[IBIS Ver]   3.2
[Comment Char]   |_char
[File Name]   sprm301.ibs
[File Rev]   1.0
[Date]   November 15, 2006
[Source]   From Ansoft Q3D ver 7.0 result.
[Notes]
[Disclaimer]
[Copyright]
[Component]   F28044PZ
[Manufacturer]   ti
[Package]
| variable   typ   min   max
R_pkg   2.03359e-001  1.85676e-001  2.33646e-001
L_pkg   4.42275e-009  3.91388e-009  5.16902e-009
C_pkg   6.90400e-013  6.03899e-013  7.98201e-013
[Pin]  signal_name   model_name   R_pin   L_pin   C_pin
01   GP_IO[12]  BC3350AFHYPU_3P3PU   2.16292E-01  4.84246E-09  7.01525E-13
02   VSS   NC   2.05669E-01  4.59853E-09  7.81026E-13
03   VDDIO   NC   2.14427E-01  4.64717E-09  7.53822E-13
04   GP_IO[29]  BC3325CFHYPU_3P3PU   2.26264E-01  4.68911E-09  7.55451E-13
05   GP_IO[33]  BC3350AFHYPU_3P3PU   2.15510E-01  4.52774E-09  7.45637E-13
06   GP_IO[30]  BC3325CFHYPU_3P3PU   2.05271E-01  4.36673E-09  7.14612E-13
07   GP_IO[31]  BC3325CFHYPU_3P3PU   2.01452E-01  4.28833E-09  6.88677E-13
08   GP_IO[14]  BC3350AFHYPU_3P3PU   1.93969E-01  4.17968E-09  6.67444E-13
09   GP_IO[15]  BC3350AFHYPU_3P3PU   1.92673E-01  4.14893E-09  6.50213E-13
10   VDD   NC   1.88856E-01  4.10765E-09  6.26914E-13
11   VSS   NC   1.92989E-01  4.13681E-09  6.03899E-13
12   VDD1   NC   2.13333E-01  4.32411E-09  6.20891E-13
13   VSS1   NC   2.06448E-01  4.25241E-09  6.31248E-13
14   VSSA2   NC   2.00063E-01  4.20609E-09  6.23019E-13
15   VDDAFL2   NC   1.93798E-01  4.16585E-09  6.28937E-13
16   ADCINA[7]   NC   1.89234E-01  4.18448E-09  6.36262E-13
17   ADCINA[6]   NC   1.87412E-01  4.23464E-09  6.46472E-13
18   ADCINA[5]   NC   1.86137E-01  4.27562E-09  6.59873E-13
19   ADCINA[4]   NC   1.85769E-01  4.34569E-09  6.75681E-13
20   ADCINA[3]   NC   1.87173E-01  4.42449E-09  6.94435E-13
21   ADCINA[2]   NC   1.89523E-01  4.53444E-09  7.11496E-13
22   ADCINA[1]   NC   1.93470E-01  4.65439E-09  7.32914E-13
23   ADCINA[0]   NC   1.96936E-01  4.78656E-09  7.54045E-13
24   ADCLO   NC   2.02141E-01  4.91416E-09  7.75388E-13
25   VSSA11   NC   2.06429E-01  5.12034E-09  6.92931E-13
26   VDDAFL11   NC   2.05491E-01  4.95382E-09  6.92435E-13
27   ADCINB[0]   NC   2.00858E-01  4.71178E-09  7.76728E-13
28   ADCINB[1]   NC   1.94857E-01  4.55615E-09  7.54959E-13
29   ADCINB[2]   NC   1.92781E-01  4.41548E-09  7.34283E-13
30   ADCINB[3]   NC   1.88419E-01  4.26915E-09  7.14862E-13
31   ADCINB[4]   NC   1.86413E-01  4.13080E-09  6.95435E-13
32   ADCINB[5]   NC   1.85676E-01  4.05447E-09  6.78346E-13
33   ADCINB[6]   NC   1.86563E-01  3.97672E-09  6.63340E-13
34   ADCINB[7]   NC   1.88600E-01  3.93329E-09  6.49418E-13
35   ADCREFIN   NC   1.91978E-01  3.91388E-09  6.38953E-13
36   ADCREFM   NC   1.97273E-01  3.93821E-09  6.32494E-13
37   ADCREFP   NC   2.04030E-01  4.00314E-09  6.29101E-13
38   ADCRESEXT   NC   2.12412E-01  4.05794E-09  6.41591E-13
39   VSSA1   NC   2.20295E-01  4.17640E-09  6.49431E-13
40   VDDA1   NC   2.26915E-01  4.30270E-09  6.53434E-13
41   VSS   NC   2.25777E-01  4.36227E-09  6.44913E-13
42   VDD   NC   2.09612E-01  4.25306E-09  6.56261E-13
43   GP_IO[34]  BC3350AFHYPU_3P3PU   2.17167E-01  4.40172E-09  6.83134E-13
44   GP_IO[1]   BC3350AFHYPU_3P3PU   2.19379E-01  4.51534E-09  6.94421E-13
45   GP_IO[2]   BC3350AFHYPU_3P3PU   2.16721E-01  4.56076E-09  7.15544E-13
46   VDDIO   NC   2.26017E-01  4.78354E-09  7.35852E-13
47   GP_IO[0]   BC3350AFHYPU_3P3PU   2.11005E-01  4.69198E-09  7.46315E-13
48   GP_IO[3]   BC3350AFHYPU_3P3PU   2.21106E-01  4.92036E-09  7.83494E-13
49   VSS   NC   2.33646E-01  5.16902E-09  7.98201E-13
50   GP_IO[16] BC3350AFHYPU_3P3PU   2.13744E-01  5.12910E-09  6.84259E-13
51   GP_IO[4]  BC3350AFHYPU_3P3PU   2.26398E-01  4.92342E-09  7.06407E-13
52   GP_IO[17] BC3350AFHYPU_3P3PU   2.15844E-01  4.68935E-09  7.95814E-13
53   GP_IO[5]  BC3350AFHYPU_3P3PU   2.04033E-01  4.50014E-09  7.72035E-13
54   GP_IO[18] BC3350AFHYPU_3P3PU   1.95635E-01  4.36218E-09  7.46249E-13
55   VSS   NC   1.89527E-01  4.27092E-09  7.11302E-13
56   GP_IO[6]  BC3350AFHYPU_3P3PU   1.96559E-01  4.26988E-09  6.97016E-13
57   GP_IO[19] BC3350AFHYPU_3P3PU   1.91406E-01  4.17811E-09  6.85500E-13
58   GP_IO[7]  BC3350AFHYPU_3P3PU   1.87512E-01  4.10710E-09  6.64382E-13
59   VDD   NC   1.85845E-01  4.07460E-09  6.37606E-13
60   GP_IO[8]  BC3350AFHYPU_3P3PU   1.88779E-01  4.07856E-09  6.23034E-13
61   GP_IO[9]  BC3350AFHYPU_3P3PU   1.86926E-01  4.03716E-09  6.20859E-13
62   VSS   NC   1.86440E-01  4.04566E-09  6.02703E-13
63   GP_IO[20] BC3350AFHYPU_3P3PU   1.88373E-01  4.05495E-09  6.04095E-13
64   GP_IO[10] BC3350AFHYPU_3P3PU   1.88009E-01  4.08425E-09  6.12057E-13
65   VDDIO   NC   1.85978E-01  4.10911E-09  6.20487E-13
66   XCLKOUT   BC3325CF_3P3PU   1.86925E-01  4.17194E-09  6.25512E-13
67   GP_IO[21] BC3350AFHYPU_3P3PU   1.86819E-01  4.21956E-09  6.40861E-13
68   VDD   NC   1.89866E-01  4.31866E-09  6.54786E-13
69   VSS   NC   1.85610E-01  4.34307E-09  6.58781E-13
70   GP_IO[11] BC3350AFHYPU_3P3PU   1.86090E-01  4.36372E-09  6.88671E-13
71   GP_IO[22] BC3350AFHYPU_3P3PU   1.86568E-01  4.45206E-09  7.16155E-13
72   GP_IO[23] BC3350AFHYPU_3P3PU   1.87669E-01  4.56253E-09  7.38219E-13
73   TDI   IC33FFSHYPU_3P3PU   1.93987E-01  4.72336E-09  7.60132E-13
74   TMS   IC33FFSHYPU_3P3PU   2.01048E-01  4.88251E-09  7.86418E-13
75   TCK   IC33FFSHYPU_3P3PU   2.11249E-01  5.18088E-09  7.03348E-13
76   TDO   OC3325CF_3P3   2.06688E-01  4.94914E-09  6.96076E-13
77   VSS   NC   1.98342E-01  4.65382E-09  7.80676E-13
78   XRSn   BC3350BFODHYPU_3P3PU   1.93176E-01  4.48692E-09  7.57321E-13
79   GP_IO[27] BC3350AFHYPU_3P3PU   1.88188E-01  4.31589E-09  7.28548E-13
80   EMU0   BC3325CFHYPU_3P3PU   1.89619E-01  4.26207E-09  7.10142E-13
81   EMU1   BC3325CFHYPU_3P3PU   1.86922E-01  4.12139E-09  6.97582E-13
82   VDDIO   NC   1.85269E-01  4.01949E-09  6.82524E-13
83   GP_IO[24] BC3350AFHYPU_3P3PU   1.85832E-01  3.93920E-09  6.64624E-13
84   TRSTn   IC33FFSHYPD_3P3PD   1.87384E-01  3.90020E-09  6.46879E-13
85   VDD   NC   1.90176E-01  3.87909E-09  6.26008E-13
86   X2   NC   1.85448E-01  3.83198E-09  6.08398E-13
87   VSS   NC   1.87288E-01  3.82154E-09  6.08983E-13
88   X1   NC   1.89799E-01  3.81436E-09  6.13885E-13
89   VSS   NC   1.91602E-01  3.87476E-09  6.15372E-13
90   XCLKIN   BC3350AFHYPU_3P3PU   1.95306E-01  3.94123E-09  6.27780E-13
91   GP_IO[25] BC3350AFHYPU_3P3PU   1.99443E-01  4.04240E-09  6.37161E-13
92   GP_IO[28] BC3325CFHYPU_3P3PU   2.03022E-01  4.16398E-09  6.48097E-13
93   VDD   NC   2.00114E-01  4.20193E-09  6.56967E-13
94   VSS   NC   1.90892E-01  4.16295E-09  6.61041E-13
95   GP_IO[13] BC3350AFHYPU_3P3PU   1.86615E-01  4.16393E-09  6.81384E-13
96   VDD3V   NC   1.84802E-01  4.25057E-09  7.10450E-13
97   TEST1   NC   1.88155E-01  4.37973E-09  7.37857E-13
98   TEST2   NC   1.91621E-01  4.56227E-09  7.56701E-13
99   GP_IO[18] BC3350AFHYPU_3P3PU   1.97169E-01  4.74011E-09  7.77284E-13
100   GP_IO[18] BC3350AFHYPU_3P3PU   2.04213E-01  5.01635E-09  6.90838E-13
[Define Package Model]  pz_dd6_1
[Manufacturer]   ti
[OEM]   xyz
[Description]  None
[Number Of Pins]  100
[Pin Numbers]
01   | 01 = P001
02   | 02 = P002
03   | 03 = P003
04   | 04 = P004
05   | 05 = P005
06   | 06 = P006
07   | 07 = P007
08   | 08 = P008
09   | 09 = P009
10   | 10 = P010
11   | 11 = P011
12   | 12 = P012
13   | 13 = P013
14   | 14 = P014
15   | 15 = P015
16   | 16 = P016
17   | 17 = P017
18   | 18 = P018
19   | 19 = P019
20   | 20 = P020
21   | 21 = P021
22   | 22 = P022
23   | 23 = P023
24   | 24 = P024
25   | 25 = P025
26   | 26 = P026
27   | 27 = P027
28   | 28 = P028
29   | 29 = P029
30   | 30 = P030
31   | 31 = P031
32   | 32 = P032
33   | 33 = P033
34   | 34 = P034
35   | 35 = P035
36   | 36 = P036
37   | 37 = P037
38   | 38 = P038
39   | 39 = P039
40   | 40 = P040
41   | 41 = P041
42   | 42 = P042
43   | 43 = P043
44   | 44 = P044
45   | 45 = P045
46   | 46 = P046
47   | 47 = P047
48   | 48 = P048
49   | 49 = P049
50   | 50 = P050
51   | 51 = P051
52   | 52 = P052
53   | 53 = P053
54   | 54 = P054
55   | 55 = P055
56   | 56 = P056
57   | 57 = P057
58   | 58 = P058
59   | 59 = P059
60   | 60 = P060
61   | 61 = P061
62   | 62 = P062
63   | 63 = P063
64   | 64 = P064
65   | 65 = P065
66   | 66 = P066
67   | 67 = P067
68   | 68 = P068
69   | 69 = P069
70   | 70 = P070
71   | 71 = P071
72   | 72 = P072
73   | 73 = P073
74   | 74 = P074
75   | 75 = P075
76   | 76 = P076
77   | 77 = P077
78   | 78 = P078
79   | 79 = P079
80   | 80 = P080
81   | 81 = P081
82   | 82 = P082
83   | 83 = P083
84   | 84 = P084
85   | 85 = P085
86   | 86 = P086
87   | 87 = P087
88   | 88 = P088
89   | 89 = P089
90   | 90 = P090
91   | 91 = P091
92   | 92 = P092
93   | 93 = P093
94   | 94 = P094
95   | 95 = P095
96   | 96 = P096
97   | 97 = P097
98   | 98 = P098
99   | 99 = P099
100   | 100 = P100
[Model Data]
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[End Model Data]
[End Package Model]
|   Component BC3350AFHYPU
[Component]   BC3350AFHYPU
[Manufacturer]   Texas Instruments.
[Package]
| variable   typ   min   max
R_pkg   0.000   0.000   0.000
L_pkg   0.000H   0.000H   0.000H
C_pkg   0.000F   0.000F   0.000F
[Pin]  signal_name   model_name   R_pin   L_pin   C_pin
PAD   PAD   BC3350AFHYPU_3P3PU
| A   A   dummy
| GZ   GZ   dummy
| Y   Y   dummy
VSSS   VSSS   GND
VDDS   VDDS   POWER
[Model Selector]  BC3350AFHYPU
BC3350AFHYPU_2P5PU   cell   VDDS=2.5V(typ)  PI=0
BC3350AFHYPU_2P5PUZ  cell   VDDS=2.5V(typ)  PI=1
BC3350AFHYPU_3P3PU   cell   VDDS=3.3V(typ)  PI=0
BC3350AFHYPU_3P3PUZ  cell   VDDS=3.3V(typ)  PI=1
|   Component BC3325CFHYPU
[Component]   BC3325CFHYPU
[Manufacturer]   Texas Instruments.
[Package]
| variable   typ   min   max
R_pkg   0.000   0.000   0.000
L_pkg   0.000H   0.000H   0.000H
C_pkg   0.000F   0.000F   0.000F
[Pin]  signal_name   model_name   R_pin   L_pin   C_pin
PAD   PAD   BC3325CFHYPU_3P3PU
| A   A   dummy
| GZ   GZ   dummy
| Y   Y   dummy
VSSS   VSSS   GND
VDDS   VDDS   POWER
[Model Selector]   BC3325CFHYPU
BC3325CFHYPU_2P5PU   cell  VDDS=2.75(TYP)  PI=0
BC3325CFHYPU_2P5PUZ   cell  VDDS=2.75(TYP)  PI=1
BC3325CFHYPU_3P3PU   cell  VDDS=3.3(TYP)  PI=0
BC3325CFHYPU_3P3PUZ   cell  VDDS=3.3(TYP)  PI=1
|   Component OC3325CF
[Component]   OC3325CF
[Manufacturer]   Texas Instruments.
[Package]
| variable   typ   min   max
R_pkg   0.000   0.000   0.000
L_pkg   0.000H   0.000H   0.000H
C_pkg   0.000F   0.000F   0.000F
[Pin]  signal_name   model_name   R_pin   L_pin   C_pin
PAD   PAD   OC3325CF_3P3
| A   A   dummy
| GZ   GZ   dummy
VDDS   VDDS   POWER
VSSS   VSSS   GND
VSS   VSS   GND
[Model Selector]   OC3325CF
OC3325CF_2P5  cell VDDS=2.5V(typ)
OC3325CF_2P7  cell VDDS=2.75V(typ)
OC3325CF_3P3  cell VDDS=3.3V(typ)
|   Component BC3350BFODHYPU
[Component]   BC3350BFODHYPU
[Manufacturer]   Texas Instruments.
[Package]
| variable   typ   min   max
R_pkg   0.000   0.000   0.000
L_pkg   0.000H   0.000H   0.000H
C_pkg   0.000F   0.000F   0.000F
[Pin]  signal_name   model_name   R_pin   L_pin   C_pin
PAD   PAD   BC3350BFODHYPU_3P3PU
| A   A   dummy
| GZ   GZ   dummy
| Y   Y   dummy
VSSS   VSSS   GND
VDDS   VDDS   POWER
[Model Selector]   BC3350BFODHYPU
BC3350BFODHYPU_2P5PU   cell   VDDS=2.75(TYP)
BC3350BFODHYPU_2P5PZ   cell   VDDS=2.75(TYP)
BC3350BFODHYPU_3P3PU   cell   VDDS=3.3(TYP)
BC3350BFODHYPU_3P3PZ   cell   VDDS=3.3(TYP)
|   Component IC33FFSHYPD
[Component]   IC33FFSHYPD
[Manufacturer]   Texas Instruments.
[Package]
| variable   typ   min   max
R_pkg   0.000   0.000   0.000
L_pkg   0.000H   0.000H   0.000H
C_pkg   0.000F   0.000F   0.000F
[Pin]  signal_name   model_name   R_pin   L_pin   C_pin
PAD   PAD   IC33FFSHYPD_3P3PD
| Y   Y   dummy
VSS   VSS   GND
VDDS   VDDS   POWER
[Model Selector]  IC33FFSHYPD
IC33FFSHYPD_2P7PD   cell with PI=0 and VDDS as 2.75(typ)
IC33FFSHYPD_2P7PDZ   cell with PI=1 and VDDS as 2.75(typ)
IC33FFSHYPD_3P3PD   cell with PI=0 and VDDS as 3.3(typ)
IC33FFSHYPD_3P3PDZ   cell with PI=1 and VDDS as 3.3(typ)
|   Component BC3325CF
[Component]   BC3325CF
[Manufacturer]   Texas Instruments.
[Package]
| variable   typ   min   max
R_pkg   0.000   0.000   0.000
L_pkg   0.000H   0.000H   0.000H
C_pkg   0.000F   0.000F   0.000F
[Pin]  signal_name   model_name   R_pin   L_pin   C_pin
PAD   PAD   BC3325CF_3P3PU
| A   A   dummy
| GZ   GZ   dummy
| Y   Y   dummy
VSSS   VSSS   GND
VDDS   VDDS   POWER
[Model Selector]  BC3325CF
BC3325CF_2P5PU  cell   VDDS=2.75V(typ)
BC3325CF_3P3PU  cell   VDDS=3.30V(typ)
|   Component IC33FFSHYPU
[Component]   IC33FFSHYPU
[Manufacturer]   Texas Instruments.
[Package]
| variable   typ   min   max
R_pkg   0.000   0.000   0.000
L_pkg   0.000H   0.000H   0.000H
C_pkg   0.000F   0.000F   0.000F
[Pin]  signal_name   model_name   R_pin   L_pin   C_pin
PAD   PAD   IC33FFSHYPU_3P3PU
| Y   Y   dummy
VSS   VSS   GND
VDDS   VDDS   POWER
[Model Selector]  IC33FFSHYPU
IC33FFSHYPU_2P5PU   cell with PI=0 VDDS=2.5(typ)
IC33FFSHYPU_2P5PUZ   cell with PI=1 VDDS=2.5(typ)
IC33FFSHYPU_2P7PU   cell with PI=0 VDDS=2.7(typ)
IC33FFSHYPU_2P7PUZ   cell with PI=1 VDDS=2.7(typ)
IC33FFSHYPU_3P3PU   cell with PI=0 VDDS=3.3(typ)
IC33FFSHYPU_3P3PUZ   cell with PI=1 VDDS=3.3(typ)
| Models and submodels in the file (27): BC3350AFHYPU_2P5PU (I/O), BC3350AFHYPU_2P5PUZ (I/O), BC3350AFHYPU_3P3PU (I/O), BC3350AFHYPU_3P3PUZ (I/O), BC3325CFHYPU_2P5PU (I/O), BC3325CFHYPU_2P5PUZ (I/O), BC3325CFHYPU_3P3PU (I/O), BC3325CFHYPU_3P3PUZ (I/O), OC3325CF_2P5 (3-state), OC3325CF_2P7 (3-state), OC3325CF_3P3 (3-state), BC3350BFODHYPU_2P5PU (I/O_open_drain), BC3350BFODHYPU_2P5PZ (I/O_open_drain), BC3350BFODHYPU_3P3PU (I/O_open_drain), BC3350BFODHYPU_3P3PZ (I/O_open_drain), IC33FFSHYPD_2P7PD (Input), IC33FFSHYPD_2P7PDZ (Input), IC33FFSHYPD_3P3PD (Input), IC33FFSHYPD_3P3PDZ (Input), BC3325CF_2P5PU (I/O), BC3325CF_3P3PU (I/O), IC33FFSHYPU_2P5PU (Input), IC33FFSHYPU_2P5PUZ (Input), IC33FFSHYPU_2P7PU (Input), IC33FFSHYPU_2P7PUZ (Input), IC33FFSHYPU_3P3PU (Input), IC33FFSHYPU_3P3PUZ (Input)
